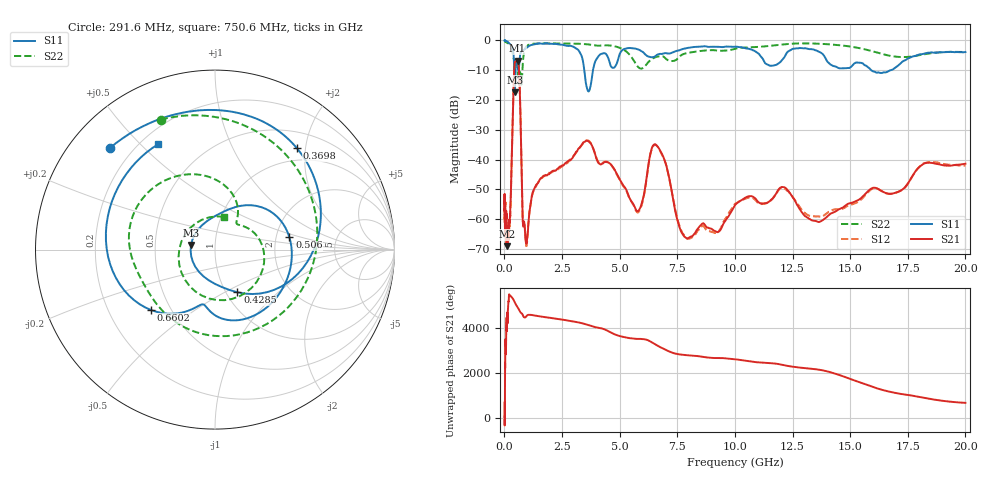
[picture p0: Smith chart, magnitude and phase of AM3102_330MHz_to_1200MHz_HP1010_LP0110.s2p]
! Date/Time: Tue, Sep 11, 2018 5:19 PM
! Network Analyzer: Agilent Technologies E8362B Rev: A.07.50.63
! Sweep from 0.010 to 20.000 GHz, 1601 Points, Sweep Type: LOG
! Power Supply: 4.949 V, 0.001 A
# Hz S DB R 50
!freq MagS11 AngS11 MagS21 AngS21 MagS12 AngS12 MagS22 AngS22
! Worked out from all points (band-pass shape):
!   1601 points, 10 MHz to 20 GHz, reference 50 ohm
!   highest |S21| = -6.81 dB at 572.5 MHz (marker M1); lowest = -69.0 dB at 126.4 MHz (marker M2)
!   |S21| within 3 dB of the highest: 427.1 MHz to 632.4 MHz (205.3 MHz wide, 38.7 % of centre)
!   lowest |S11| = -17.3 dB at 451.5 MHz (marker M3), VSWR 1.31, Z = 38.2 + j2.02 ohm
!   |S11| at or under -10 dB: 425 MHz to 479.8 MHz (54.86 MHz wide, 12.1 % of centre); 3.468 GHz to 3.842 GHz (374.8 MHz wide, 10.3 % of centre); 15.92 GHz to 16.76 GHz (839.5 MHz wide, 5.14 % of centre)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
!   |S22| runs from -14.8 to -0.2 dB; largest |S21 - S12| = 0.008
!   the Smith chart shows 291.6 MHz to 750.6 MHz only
!   S11 on the Smith chart (normalised r, x): 291.6 MHz: 0.12, +0.40; 369.8 MHz: 0.77, +1.84; 428.5 MHz: 1.13, -0.58; 506 MHz: 2.37, +0.40; 660.2 MHz: 0.39, -0.34; 750.6 MHz: 0.27, +0.57
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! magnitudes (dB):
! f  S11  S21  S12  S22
! 10 MHz  0.0  -51.8  -61.2  -0.2
! 35.55 MHz  0.0  -63.3  -62.9  -0.3
! 126.4 MHz  -0.4  -69.0  -64.5  -0.8
! 177.9 MHz  -0.7  -65.1  -66.4  -1.0
! 291.6 MHz  -1.8  -48.1  -48.4  -2.1
! 369.8 MHz  -2.8  -23.7  -23.8  -4.9
! 428.5 MHz  -11.4  -9.6  -9.7  -6.9
! 447.2 MHz  -17.2  -7.8  -7.8  -7.1
! 451.5 MHz  -17.3  -7.6  -7.6  -7.1
! 506 MHz  -7.5  -7.0  -7.1  -6.1
! 572.5 MHz  -8.1  -6.8  -6.9  -9.7
! 660.2 MHz  -6.2  -14.7  -14.7  -11.1
! 750.6 MHz  -3.5  -44.8  -45.0  -14.4
! 802.2 MHz  -3.4  -61.4  -60.9  -7.4
! 956.4 MHz  -2.5  -68.1  -68.9  -2.0
! 1.59 GHz  -1.1  -46.2  -46.3  -1.0
! 3.107 GHz  -2.7  -37.4  -37.6  -1.1
! 3.617 GHz  -16.8  -33.7  -33.6  -1.3
! 5.652 GHz  -2.7  -55.9  -56.1  -7.2
! 6.58 GHz  -5.1  -35.0  -35.2  -5.5
! 7.958 GHz  -2.5  -66.5  -66.5  -4.2
! 20 GHz  -3.9  -41.3  -42.0  -3.9
